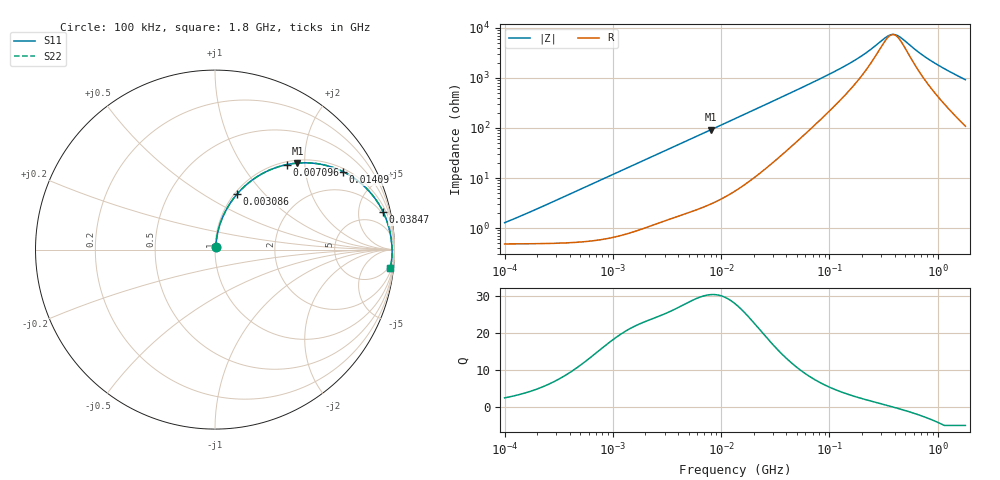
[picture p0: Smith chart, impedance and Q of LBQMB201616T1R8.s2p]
! LBQMB201616T1R8  S-PARAMETER MODEL  ( General Type )
! Model Generated by TAIYO YUDEN Corporation (http://www.ty-top.com)
! Version 1.0
! TAIYO YUDEN Control No. 191025NI43SB-FBB
! Copyright(c) 2019 TAIYO YUDEN CO.,LTD. All Rights Reserved.
! Product Description (link to TY-COMPAS)
! https://ds.yuden.co.jp/TYCOMPAS/or/detail?pn=LBQMB201616T1R8J&u=M
! Products Name : Inductors
! Characteristics :
!  Inductance : 1.8 uH , SRF(min) : 100 MHz , DC Resistance(max) : 0.624 Ohm , Rated Current : 345 mA
!  Case Size : 2.0 x 1.6 / 0.079 x 0.063 [mm/inch] , Thickness : 1.6 / 0.063 [mm/inch]
!  (Conditions: Temperature = 25 degC , DC Bias Current/Voltage = 0A / 0V)
! External Node Assignments :
!  1  o---GGG---o  2
! GND o---------o GND
! Frequency Range : 0.1MHz  -  1800MHz  [ 402 STEP ]
# MHz S RI R 50
! Freq[MHz].  S11 Real  S11 Imag  S21 Real  S21 Imag  S12 Real  S12 Imag  S22 Real  S22 Imag
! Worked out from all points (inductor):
!   401 points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, 100 kHz to 1.8 GHz, reference 50 ohm
!   read as one part in series: L = 1.89 uH near 124.7 kHz
!   highest Q = 30.4 at 8.021 MHz (marker M1), where L = 1.82 uH
!   self-resonance near 384.5 MHz
!   S11 on the Smith chart (normalised r, x): 100 kHz: 1.01, +0.02; 3.086 MHz: 1.03, +0.72; 7.096 MHz: 1.05, +1.63; 14.09 MHz: 1.12, +3.22; 38.47 MHz: 1.65, +8.80; 1.8 GHz: 3, -18
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0.1  0.00494 0.0118  0.9951 -0.0118  0.9951 -0.0118  0.00494 0.0118
0.171412  0.00524 0.0202  0.9948 -0.0202  0.9948 -0.0202  0.00524 0.0202
0.516129  0.00894 0.0604  0.9911 -0.0604  0.9911 -0.0604  0.00894 0.0604
1.216451  0.0269 0.1388  0.9731 -0.1388  0.9731 -0.1388  0.0269 0.1388
2.66389  0.0974 0.2768  0.9026 -0.2768  0.9026 -0.2768  0.0974 0.2768
3.085641  0.1236 0.3099  0.8764 -0.3099  0.8764 -0.3099  0.1236 0.3099
4.679446  0.2337 0.4056  0.7663 -0.4056  0.7663 -0.4056  0.2337 0.4056
7.096489  0.4019 0.474  0.5981 -0.474  0.5981 -0.474  0.4019 0.474
8.02111  0.4594 0.4822  0.5406 -0.4822  0.5406 -0.4822  0.4594 0.4822
10.24746  0.5764 0.4777  0.4236 -0.4777  0.4236 -0.4777  0.5764 0.4777
13.41641  0.6953 0.4427  0.3047 -0.4427  0.3047 -0.4427  0.6953 0.4427
14.09005  0.7148 0.4337  0.2852 -0.4337  0.2852 -0.4337  0.7148 0.4337
22.44079  0.8567 0.3275  0.1433 -0.3275  0.1433 -0.3275  0.8567 0.3275
38.46609  0.9374 0.2083  0.0626 -0.2083  0.0626 -0.2083  0.9374 0.2083
69.24595  0.9702 0.1176  0.0298 -0.1176  0.0298 -0.1176  0.9702 0.1176
171.3985  0.9838 0.0405  0.0162 -0.0405  0.0162 -0.0405  0.9838 0.0405
357.3983  0.9865 0.00339  0.0135 -0.00339  0.0135 -0.00339  0.9865 0.00339
394.1897  0.9867 -0.00115  0.0133 0.00115  0.0133 0.00115  0.9867 -0.00115
434.7684  0.9868 -0.00571  0.0132 0.00571  0.0132 0.00571  0.9868 -0.00571
842.3428  0.9856 -0.0406  0.0144 0.0406  0.0144 0.0406  0.9856 -0.0406
1246.522  0.9826 -0.0686  0.0174 0.0686  0.0174 0.0686  0.9826 -0.0686
1800  0.9763 -0.1039  0.0237 0.1039  0.0237 0.1039  0.9763 -0.1039
